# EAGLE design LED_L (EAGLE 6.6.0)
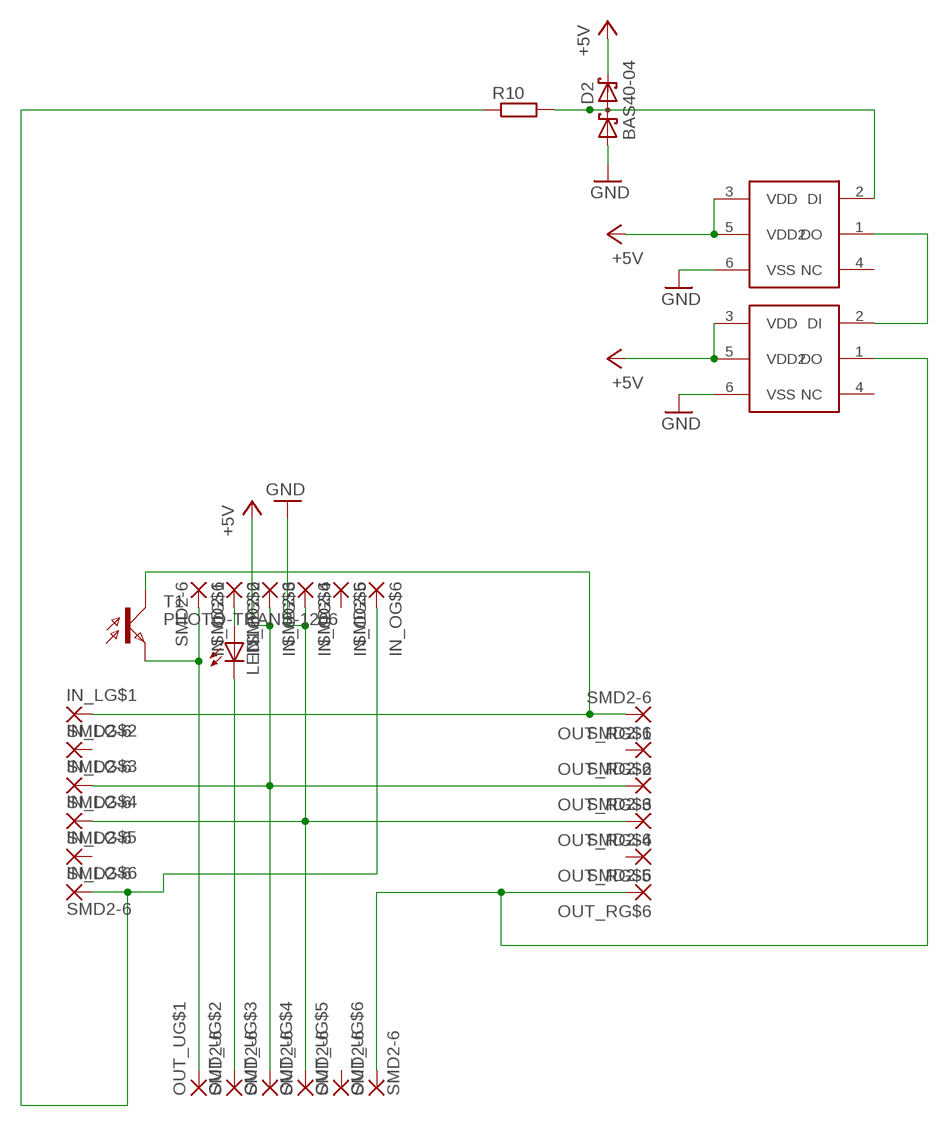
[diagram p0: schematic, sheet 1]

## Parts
D2  BAS40-04  [SOT23]
IN_L  SMD2-6  [SMD1,27-2,54-6]
IN_O  SMD2-6  [SMD1,27-2,54-6]
LED1  LED3MM  [LED3MM]
OUT_R  SMD2-6  [SMD1,27-2,54-6]
OUT_U  SMD2-6  [SMD1,27-2,54-6]
R10  R-EU_M1206  [M1206]
T1  PHOTO-TRANS-1206  [1206]
U$1  LED_SMD5050  [CLN6A]
U$2  LED_SMD5050  [CLN6A]

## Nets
+5V: D2.2(C2) IN_L.3 IN_O.3 OUT_R.3 OUT_U.3 U$1.3(VDD) U$1.5(VDD2) U$2.3(VDD) U$2.5(VDD2)
GND: D2.1(A1) IN_L.4 IN_O.4 OUT_R.4 OUT_U.4 U$1.6(VSS) U$2.6(VSS)
N$4: IN_O.1 OUT_U.1 T1.C(E)
N$6: U$1.1(DO) U$2.2(DI)
N$7: D2.3(C1A2) R10.2 U$1.2(DI)
N$13: IN_O.2 LED1.A
N$17: IN_L.6 IN_O.6 R10.1
N$18: IN_L.1 OUT_R.1 T1.A(C)
N$21: OUT_R.6 OUT_U.6 U$2.1(DO)
N$25: LED1.K(C) OUT_U.2
Unconnected: IN_L.2 IN_L.5 IN_O.5 OUT_R.2 OUT_R.5 OUT_U.5 U$1.4(NC) U$2.4(NC)

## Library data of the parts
D2 = diode:BAS40-04: Silicon Schottky Diodes General-purpose diode for high-speed switching
IN_L IN_O OUT_R OUT_U = #mylib:SMD2-6
LED1 = led:LED: LED
R10 = resistor:R-EU_: RESISTOR, European symbol
T1 = #mylib:PHOTO-TRANS-1206: PHOTO TRANSISTOR
U$1 U$2 = #mylib:LED_SMD5050

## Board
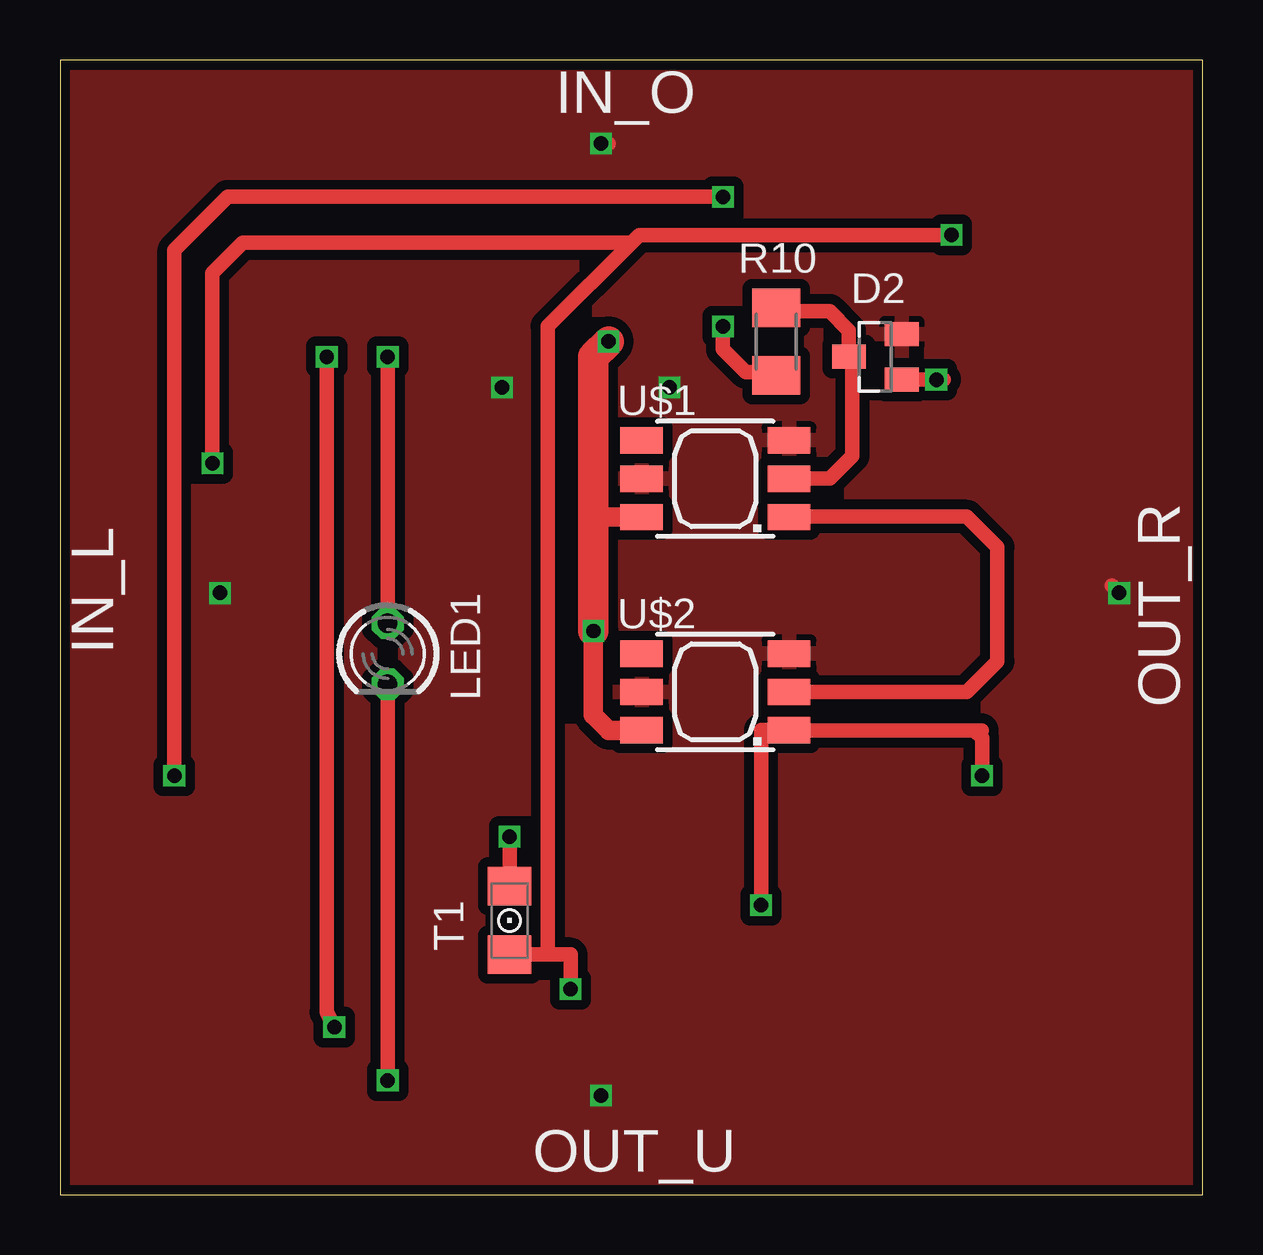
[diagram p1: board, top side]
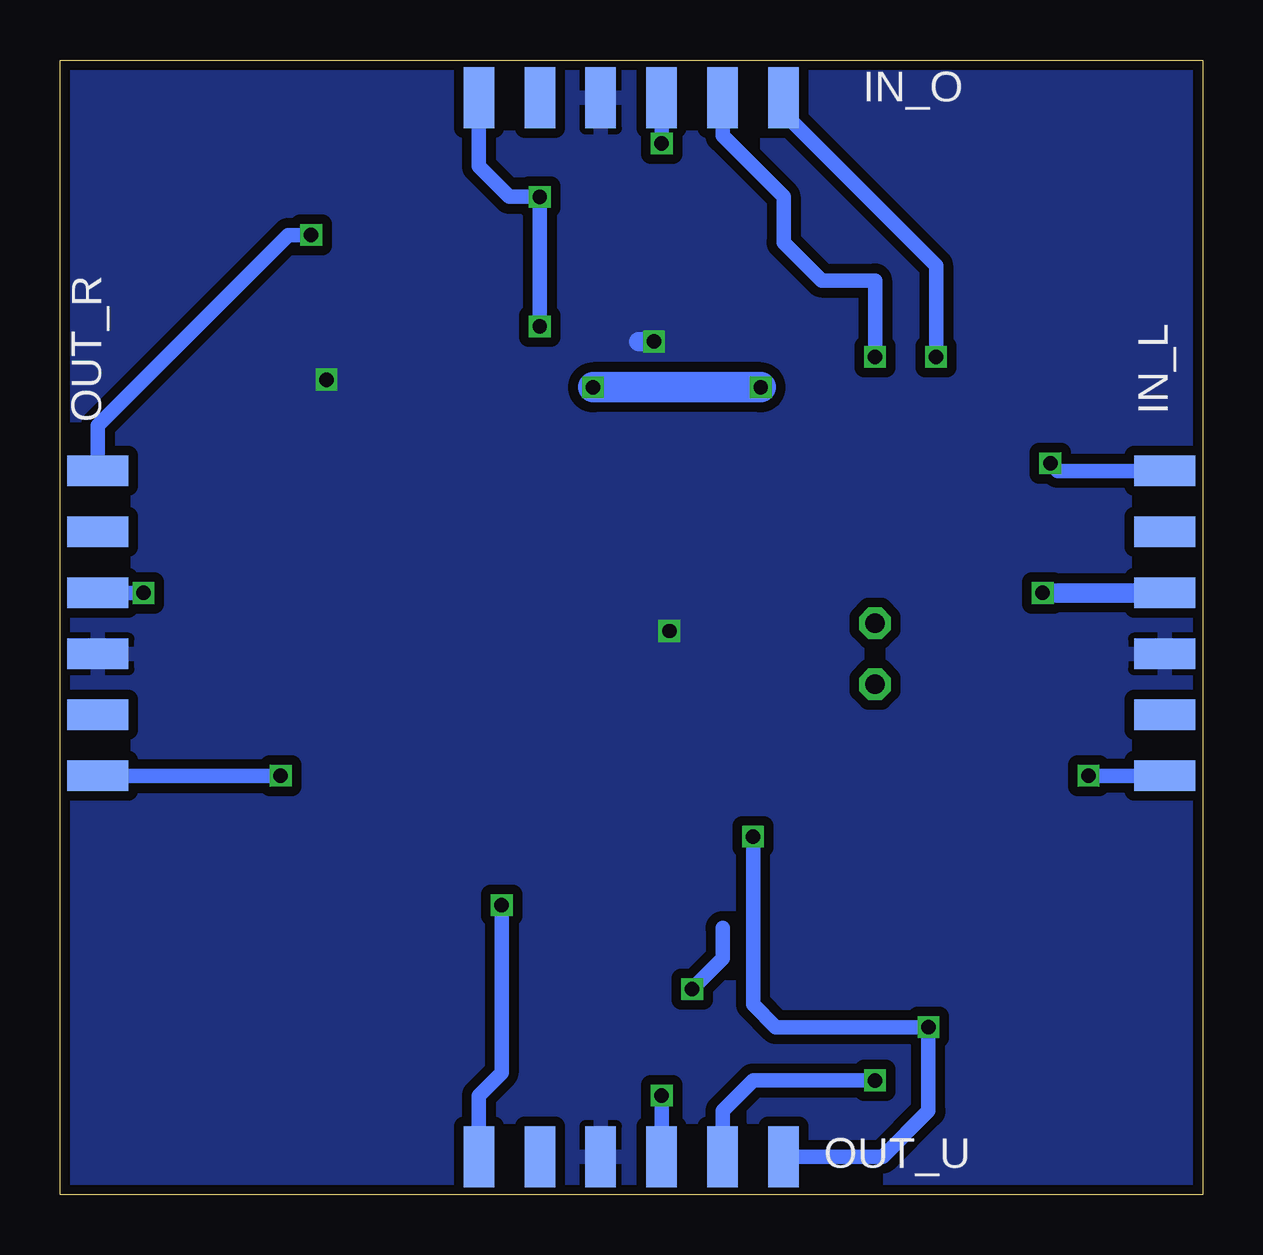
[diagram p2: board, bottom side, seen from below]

Size 47.61 x 47.3 mm. Coordinates in mm from the lower left corner, seen from the top.
Outline: 0,0 47.61,0 47.61,47.3 0,47.3 0,0
Copper layers (1*16): Top 0.035mm / dielectric 1.5mm / Bottom 0.035mm
Design rules "Elecrow_2-layer_eagle_rule": minimum track width 6mil, minimum drill 12mil, track to track 6mil, track to pad 6mil, pad to pad 6mil, via to via 6mil, smd to smd 0mil, copper to edge 10mil, drill to drill 10mil, minimum pad ring 10mil, minimum via ring 6mil, stop-mask expansion 2mil, vias tented up to drill 100mil, thermal gap 10mil

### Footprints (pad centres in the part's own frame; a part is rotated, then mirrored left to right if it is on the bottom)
SOT23 = smd 1 x 1.4: 1 -0.95,-1.1; 2 0.95,-1.1; 3 0,1.1
SMD1,27-2,54-6 = smd 1.27 x 2.54: 1 0,0; 2 2.54,0; 3 5.08,0; 4 7.62,0; 5 10.16,0; 6 12.7,0
LED3MM = drill 0.813 octagon: A -1.27,0; K 1.27,0
M1206 = smd 1.6 x 2: 1 -1.4,0; 2 1.4,0
1206 = smd 1.6 x 1.803: A -1.422,0; C 1.422,0
CLN6A = smd 1.778 x 1.1: 1 3.071,-1.6; 2 3.071,0; 3 3.071,1.6; 4 -3.071,1.6; 5 -3.071,0; 6 -3.071,-1.6

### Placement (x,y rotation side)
D2  33.97,34.92 90 top
IN_L  1.59,30.16 270 bottom
IN_O  17.46,45.72 180 bottom
LED1  13.65,22.54 270 top
OUT_R  46.04,30.16 270 bottom
OUT_U  17.46,1.59 180 bottom
R10  29.84,35.56 90 top
T1  18.73,11.43 90 top
U$1  27.3,29.84 0 top
U$2  27.3,20.95 0 top

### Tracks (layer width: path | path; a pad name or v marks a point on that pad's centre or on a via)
+5V  (via drill 0.6)
  Top 0.61: v22.54,43.81 22.86,43.81 | v44.13,25.08 43.81,25.4
  Bottom 0.61: IN_O.3 v22.54,43.81 | OUT_R.3 v44.13,25.08 | v22.54,4.13 OUT_U.3
  Bottom 0.813: IN_L.3 v6.67,25.08
  Bottom 1.27: v18.41,33.66 v25.4,33.66
  pour Top (isolate 0.406): 0.32,46.99 47.31,46.99 47.31,0.32 0.32,0.32
GND  (via drill 0.6)
  Top 0.61: D2.1 36.83,33.98 v36.51,33.97
  Top 0.813: U$2.6 22.87,19.36 22.23,20 v22.23,23.5 | U$1.6 22.24,28.25 22.23,28.26
  Top 1.27: v22.23,23.5 22.23,28.26 22.23,34.92 v22.86,35.56
  Bottom 0.813: v22.86,35.56 23.5,35.56
  pour Bottom (isolate 0.406): 0.32,46.99 47.31,46.99 47.31,0.32 0.32,0.32
N$4  (via drill 0.6)
  Top 0.61: v11.11,34.92 11.11,7.62 v11.43,6.99 | v18.73,14.92 T1.C
  Bottom 0.61: v11.11,34.92 11.11,38.73 17.46,45.09 IN_O.1 | v18.73,14.92 18.73,7.94 17.78,6.99 v11.43,6.99 11.43,3.49 13.34,1.59 OUT_U.1
N$6
  Top 0.61: U$2.2 37.78,20.95 39.05,22.23 39.05,26.99 37.78,28.26 30.39,28.26 U$1.1
N$7
  Top 0.61: U$1.2 32.07,29.84 33.02,30.8 33.02,34.78 D2.3 32.87,36.02 32.07,36.83 29.98,36.83 R10.2
N$13  (via drill 0.6)
  Top 0.61: v13.65,34.92 LED1.A
  Bottom 0.61: v13.65,34.92 13.65,38.1 15.88,38.1 17.46,39.69 17.46,41.59 20,44.13 IN_O.2
N$17  (via drill 0.6)
  Top 0.61: v27.62,36.2 27.62,35.24 28.57,34.29 29.71,34.29 R10.1 | v4.76,17.46 4.76,39.37 6.99,41.59 v27.62,41.59
  Bottom 0.61: v27.62,36.2 v27.62,41.59 28.89,41.59 30.16,42.86 IN_O.6 | IN_L.6 v4.76,17.46
N$18  (via drill 0.6)
  Top 0.61: v21.27,8.57 21.27,10.01 20.32,10.01 | 23.81,39.69 24.13,40.01 v37.15,40.01 | 23.81,39.69 20.32,36.2 20.32,10.01 | 20.32,10.01 T1.A | v6.35,30.48 6.35,38.42 7.62,39.69 23.81,39.69
  Bottom 0.61: 20,11.11 20,9.84 v21.27,8.57 | v37.15,40.01 38.1,40.01 46.04,32.07 OUT_R.1 | IN_L.1 6.03,30.16 v6.35,30.48
N$21  (via drill 0.6)
  Top 0.61: 38.1,19.36 U$2.1 30.38,19.37 29.21,19.37 v29.21,12.06 | 38.1,19.36 38.41,19.36 | v38.42,17.46 38.42,19.04 38.1,19.36
  Bottom 0.61: OUT_R.6 v38.42,17.46 | v29.21,12.06 29.21,5.08 30.16,4.13 OUT_U.6
N$25  (via drill 0.6)
  Top 0.61: v13.65,4.76 LED1.K
  Bottom 0.61: OUT_U.2 20,3.49 18.73,4.76 v13.65,4.76

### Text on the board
tNames: IN_O | IN_L | OUT_R | OUT_U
